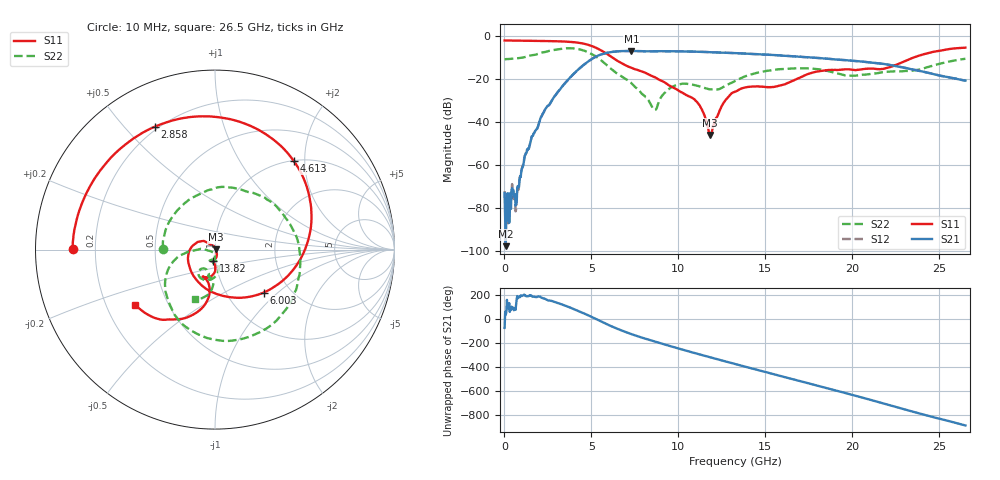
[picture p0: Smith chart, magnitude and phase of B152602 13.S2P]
!  2-Port S-parameters saved by WinCal
! VAR MeasName=S-Parameters (CALIBRATED_DATA) read from VNA (N5242A)
! VAR MeasDate=2016-1-5 16:27:15
! VAR NAME=B152602 13
! VAR FILENAME=B152602 13.S2P
! VAR DATE=2016-1-5 16:27:15
! VAR PHYS_PORTS=1,2
# Hz S DB R 50
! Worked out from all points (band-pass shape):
!   801 points, 10 MHz to 26.5 GHz, reference 50 ohm
!   highest |S21| = -6.88 dB at 7.295 GHz (marker M1); lowest = -97.6 dB at 76.22 MHz (marker M2)
!   |S21| within 3 dB of the highest: 5.173 GHz to 17.58 GHz (12.41 GHz wide, 109 % of centre)
!   lowest |S11| = -46.0 dB at 11.83 GHz (marker M3), VSWR 1.01, Z = 50.4 + j0.24 ohm
!   |S11| at or under -10 dB: 6.217 GHz to 23.5 GHz (17.29 GHz wide, 116 % of centre)
!   |S22| runs from -34.4 to -5.6 dB; largest |S21 - S12| = 0.0025
!   S11 on the Smith chart (normalised r, x): 10 MHz: 0.12, +0.00; 2.858 GHz: 0.19, +0.61; 4.613 GHz: 1.02, +1.77; 6.003 GHz: 1.48, -0.81; 13.82 GHz: 0.97, -0.12; 26.5 GHz: 0.33, -0.28
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1e7  -2.01 179.7  -72.99 -72.0  -72.02 100.4  -10.73 179.3
7.6225e7  -2.01 178.4  -97.59 39.1  -85.53 121.3  -10.71 175.1
6.7225e8  -2.07 166.2  -78.04 127.4  -80.55 149.7  -10.37 133.9
1.102712e9  -2.13 157.3  -59.10 -158.8  -59.17 -159.6  -9.87 105.8
1.566288e9  -2.18 147.6  -46.61 -165.2  -46.73 -166.4  -8.92 74.6
2.857675e9  -2.35 116.2  -28.21 145.1  -28.21 145.0  -6.40 -6.3
4.447075e9  -3.32 56.7  -14.08 56.6  -14.10 56.7  -6.42 -103.0
4.612638e9  -3.61 48.2  -12.97 46.2  -12.98 46.3  -6.82 -112.5
6.003362e9  -8.84 -41.5  -7.58 -49.2  -7.57 -49.2  -14.36 -171.0
7.29475e9  -14.71 -134.0  -6.88 -123.6  -6.89 -123.6  -21.84 177.2
8.586138e9  -18.90 162.3  -7.01 176.9  -7.01 176.9  -33.94 -136.2
8.851038e9  -20.06 153.7  -6.96 165.3  -6.96 165.2  -31.13 -94.6
9.745075e9  -24.13 138.7  -7.02 127.3  -7.03 127.3  -23.17 -96.5
1.100335e10  -30.13 123.7  -7.22 75.5  -7.23 75.6  -22.91 -114.6
1.183116e10  -45.98 28.2  -7.47 42.7  -7.45 42.6  -24.70 -106.1
1.3255e10  -25.80 -89.0  -7.88 -12.5  -7.87 -12.5  -20.85 -76.9
1.381791e10  -23.90 -100.3  -8.10 -34.3  -8.08 -34.4  -18.73 -79.0
1.557288e10  -23.50 -101.2  -8.83 -101.1  -8.83 -101.3  -15.57 -96.7
1.769208e10  -16.99 -95.0  -9.96 178.1  -9.94 178.2  -15.09 -118.5
1.981128e10  -15.41 -113.9  -11.28 97.4  -11.28 97.1  -18.37 -119.1
2.209604e10  -14.56 -101.7  -13.33 5.4  -13.28 5.2  -16.52 -104.3
2.65e10  -5.35 -145.2  -20.68 -164.7  -20.67 -165.3  -10.53 -112.3
